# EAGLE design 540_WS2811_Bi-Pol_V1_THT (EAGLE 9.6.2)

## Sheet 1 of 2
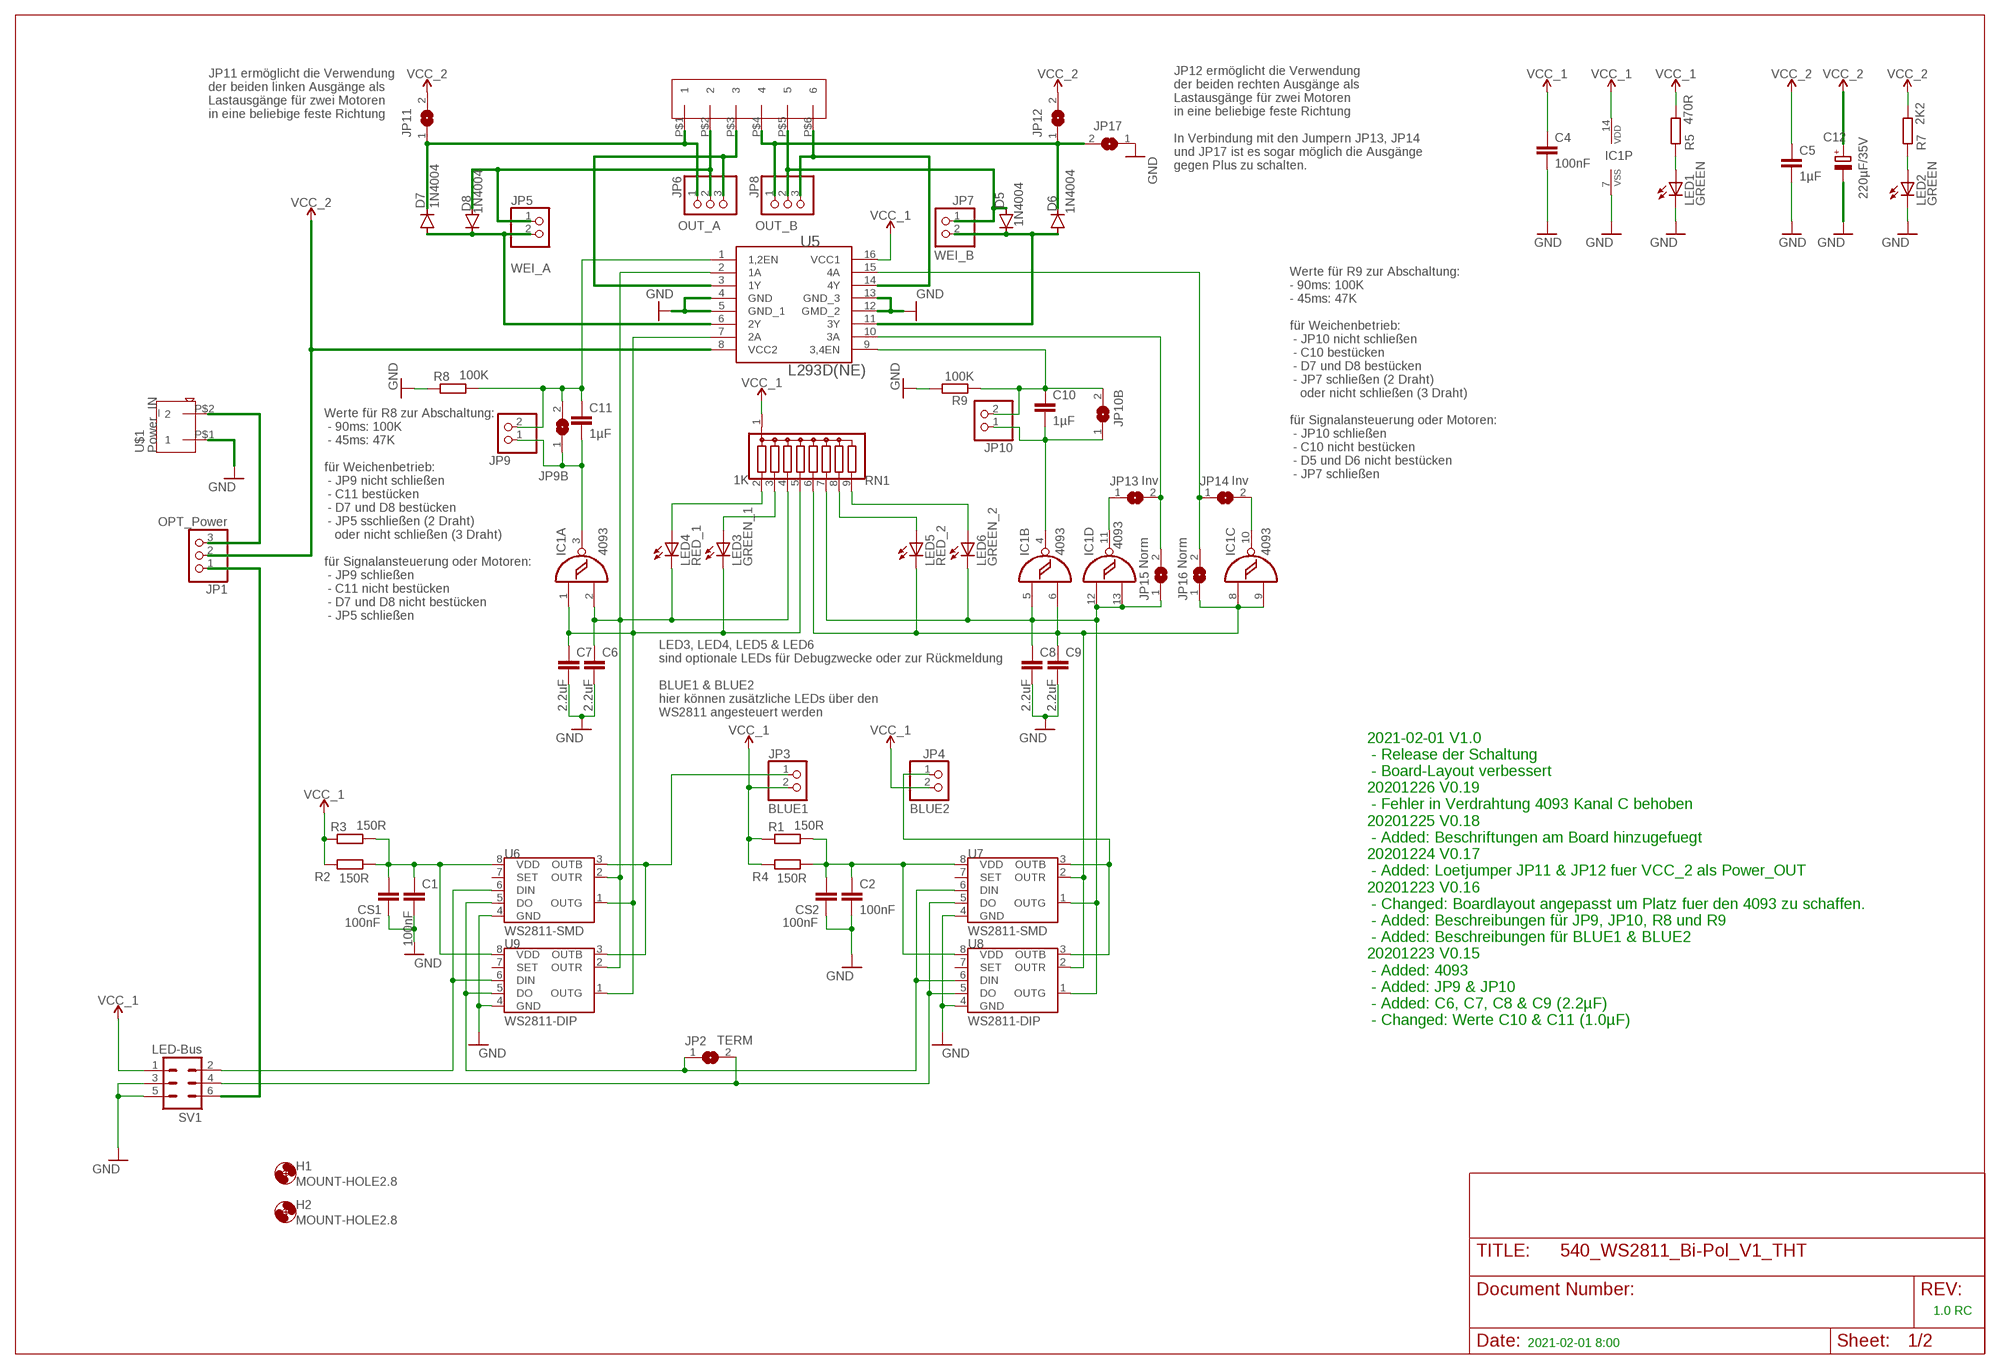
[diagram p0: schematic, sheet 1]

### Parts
C1  100nF  C-EU025-025X050  [C025-025X050]
C2  100nF  C-EU025-025X050  [C025-025X050]
C4  100nF  C-EU025-025X050  [C025-025X050]
C5  1µF  C-EU025-025X050  [C025-025X050]
C6  2.2uF  C-EU025-025X050  [C025-025X050]
C7  2.2uF  C-EU025-025X050  [C025-025X050]
C8  2.2uF  C-EU025-025X050  [C025-025X050]
C9  2.2uF  C-EU025-025X050  [C025-025X050]
C10  1µF  C-EU025-025X050  [C025-025X050]
C11  1µF  C-EU025-025X050  [C025-025X050]
C12  220µF/35V  CPOL-EUE2.5-7  [E2,5-7]
CS1  100nF  C-EUC1206  [C1206]
CS2  100nF  C-EUC1206  [C1206]
D5  1N4004  1N40041N4004-D7.5  [D-7.5]
D6  1N4004  1N40041N4004-D7.5  [D-7.5]
D7  1N4004  1N40041N4004-D7.5  [D-7.5]
D8  1N4004  1N40041N4004-D7.5  [D-7.5]
H1  MOUNT-HOLE2.8  [2,8]
H2  MOUNT-HOLE2.8  [2,8]
IC1  4093  4093N  [DIL14]
JP1  OPT_Power  PINHD-1X3  [1X03]
JP2  TERM  SJ  [SJ]
JP3  BLUE1  PINHD-1X2  [1X02]
JP4  BLUE2  PINHD-1X2  [1X02]
JP5  WEI_A  PINHD-1X2  [1X02]
JP6  OUT_A  PINHD-1X3  [1X03]
JP7  WEI_B  PINHD-1X2  [1X02]
JP8  OUT_B  PINHD-1X3  [1X03]
JP9  PINHD-1X2  [1X02]
JP9B  Inv  SJ  [SJ]
JP10  PINHD-1X2  [1X02]
JP10B  Inv  SJ  [SJ]
JP11  SJ  [SJ]
JP12  SJ  [SJ]
JP13  Inv  SJ  [SJ]
JP14  Inv  SJ  [SJ]
JP15  Norm  SJ  [SJ]
JP16  Norm  SJ  [SJ]
JP17  SJ  [SJ]
LED1  GREEN  LED3MM  [LED3MM]
LED2  GREEN  LED3MM  [LED3MM]
LED3  GREEN_1  LED3MM  [LED3MM]
LED4  RED_1  LED3MM  [LED3MM]
LED5  RED_2  LED3MM  [LED3MM]
LED6  GREEN_2  LED3MM  [LED3MM]
R1  150R  R-EU_R1206  [R1206]
R2  150R  R-EU_0207/2V  [0207/2V]
R3  150R  R-EU_R1206  [R1206]
R4  150R  R-EU_0207/2V  [0207/2V]
R5  470R  R-EU_0207/2V  [0207/2V]
R7  2K2  R-EU_0207/2V  [0207/2V]
R8  100K  R-EU_0207/2V  [0207/2V]
R9  100K  R-EU_0207/2V  [0207/2V]
RN1  1K  G08R  [SIL9]
SV1  LED-Bus  ML6  [ML6]
U5  L293D(NE)  L293DNE  [DIP-16_300MIL]
U6  WS2811-SMD  S3PO_MODUL_WS2811_SOUND_MP3-TF-16P_WS2811_AND_ATTINY_WS2811-ICSOP8  [SOP8]
U7  WS2811-SMD  S3PO_MODUL_WS2811_SOUND_MP3-TF-16P_WS2811_AND_ATTINY_WS2811-ICSOP8  [SOP8]
U8  WS2811-DIP  S3PO_MODUL_WS2811_SOUND_MP3-TF-16P_WS2811_AND_ATTINY_WS2811-ICTINY45-20-DIP  [S3PO_MODUL_WS2811_SOUND_MP3-TF-16P_WS2811_AND_ATTINY_WS2811_DIP08]
U9  WS2811-DIP  S3PO_MODUL_WS2811_SOUND_MP3-TF-16P_WS2811_AND_ATTINY_WS2811-ICTINY45-20-DIP  [S3PO_MODUL_WS2811_SOUND_MP3-TF-16P_WS2811_AND_ATTINY_WS2811_DIP08]
U$1  Power_IN  SCHRAUBKLEMME-2P  [TERM-2P]
U$2  SCHRAUBKLEMME-6P  [TERM-6P]

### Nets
GND: C1.1 C2.2 C4.2 C5.2 C6.1 C7.1 C8.1 C9.1 C12.- CS1.2 CS2.2 IC1.7(P:VSS) JP17.1 LED1.K(C) LED2.K(C) R8.1 R9.2 SV1.3 SV1.5 U5.4(GND) U5.5(GND_1) U5.12(GMD_2) U5.13(GND_3) U6.4(GND) U7.4(GND) U8.4(GND) U9.4(GND) U$1.P$1
N$1: JP1.1 SV1.6
N$2: JP1.3 U$1.P$2
N$3: C11.1 JP9.2 JP9B.2 R8.2 U5.1(1,2EN)
N$5: D6.C JP8.1 JP12.1 JP17.2 U$2.P$4
N$6: JP6.3 U5.3(1Y) U$2.P$3
N$7: D8.A JP5.1 JP6.2 U$2.P$2
N$8: JP8.3 U5.14(4Y) U$2.P$6
N$9: LED1.A R5.1
N$10: JP2.1 U6.5(DO) U7.6(DIN) U8.6(DIN) U9.5(DO)
N$11: SV1.2 U6.6(DIN) U9.6(DIN)
N$12: LED5.A RN1.8
N$13: JP3.1 U6.3(OUTB) U9.3(OUTB)
N$14: LED6.A RN1.9
N$15: C1.2 CS1.1 R2.1 R3.2 U6.8(VDD) U9.8(VDD)
N$16: JP4.1 U7.3(OUTB) U8.3(OUTB)
N$17: C2.1 CS2.1 R1.2 R4.1 U7.8(VDD) U8.8(VDD)
N$18: JP2.2 SV1.4 U7.5(DO) U8.5(DO)
N$19: C10.1 JP10.2 JP10B.2 R9.1 U5.9(3,4EN)
N$20: LED2.A R7.1
N$21: D5.C D6.A JP7.2 U5.11(3Y)
N$22: IC1.11(D:O) JP13.1
N$23: C9.2 IC1.6(B:I1) IC1.8(C:I0) IC1.9(C:I1) JP16.1 LED5.K(C) RN1.6 U7.2(OUTR) U8.2(OUTR)
N$24: C7.2 IC1.1(A:I0) LED3.K(C) RN1.5 U5.7(2A) U6.1(OUTG) U9.1(OUTG)
N$25: LED3.A RN1.3
N$26: LED4.A RN1.2
N$27: C6.2 IC1.2(A:I1) LED4.K(C) RN1.4 U5.2(1A) U6.2(OUTR) U9.2(OUTR)
N$28: D7.C JP6.1 JP11.1 U$2.P$1
N$29: D7.A D8.C JP5.2 U5.6(2Y)
N$30: C10.2 IC1.4(B:O) JP10.1 JP10B.1
N$31: D5.A JP7.1 JP8.2 U$2.P$5
N$32: C11.2 IC1.3(A:O) JP9.1 JP9B.1
N$33: C8.2 IC1.5(B:I0) IC1.12(D:I0) IC1.13(D:I1) JP15.1 LED6.K(C) RN1.7 U7.1(OUTG) U8.1(OUTG)
N$34: IC1.10(C:O) JP14.2
N$35: JP14.1 JP16.2 U5.15(4A)
N$36: JP13.2 JP15.2 U5.10(3A)
VCC_1: C4.1 IC1.14(P:VDD) JP3.2 JP4.2 R1.1 R2.2 R3.1 R4.2 R5.2 RN1.1 SV1.1 U5.16(VCC1)
VCC_2: C5.1 C12.+ JP1.2 JP11.2 JP12.2 R7.2 U5.8(VCC2)
Unconnected: U6.7(SET) U7.7(SET) U8.7(SET) U9.7(SET)

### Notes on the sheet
- JP11 ermöglicht die Verwendung 
  der beiden linken Ausgänge als
  Lastausgänge für zwei Motoren 
  in eine beliebige feste Richtung
- JP12 ermöglicht die Verwendung 
  der beiden rechten Ausgänge als
  Lastausgänge für zwei Motoren 
  in eine beliebige feste Richtung
  
  In Verbindung mit den Jumpern JP13, JP14
  und JP17 ist es sogar möglich die Ausgänge
  gegen Plus zu schalten.
- Werte für R9 zur Abschaltung:
  - 90ms: 100K
  - 45ms: 47K
  
  für Weichenbetrieb: 
   - JP10 nicht schließen
   - C10 bestücken
   - D7 und D8 bestücken
   - JP7 schließen (2 Draht) 
     oder nicht schließen (3 Draht)
  
  für Signalansteuerung oder Motoren: 
   - JP10 schließen
   - C10 nicht bestücken
   - D5 und D6 nicht bestücken
   - JP7 schließen
- Werte für R8 zur Abschaltung:
   - 90ms: 100K
   - 45ms: 47K
  
  für Weichenbetrieb: 
   - JP9 nicht schließen
   - C11 bestücken
   - D7 und D8 bestücken
   - JP5 sschließen (2 Draht) 
     oder nicht schließen (3 Draht)
  
  für Signalansteuerung oder Motoren: 
   - JP9 schließen
   - C11 nicht bestücken
   - D7 und D8 nicht bestücken
   - JP5 schließen
- LED3, LED4, LED5 & LED6 
  sind optionale LEDs für Debugzwecke oder zur Rückmeldung
  
  BLUE1 & BLUE2
  hier können zusätzliche LEDs über den
  WS2811 angesteuert werden
- 2021-02-01 V1.0
   - Release der Schaltung
   - Board-Layout verbessert
  20201226 V0.19
   - Fehler in Verdrahtung 4093 Kanal C behoben
  20201225 V0.18
   - Added: Beschriftungen am Board hinzugefuegt
  20201224 V0.17
   - Added: Loetjumper JP11 & JP12 fuer VCC_2 als Power_OUT
  20201223 V0.16
   - Changed: Boardlayout angepasst um Platz fuer den 4093 zu schaffen.
   - Added: Beschreibungen für JP9, JP10, R8 und R9
   - Added: Beschreibungen für BLUE1 & BLUE2
  20201223 V0.15
   - Added: 4093
   - Added: JP9 & JP10
   - Added: C6, C7, C8 & C9 (2.2µF)
   - Changed: Werte C10 & C11 (1.0µF)
- 1.0 RC
- 2021-02-01 8:00

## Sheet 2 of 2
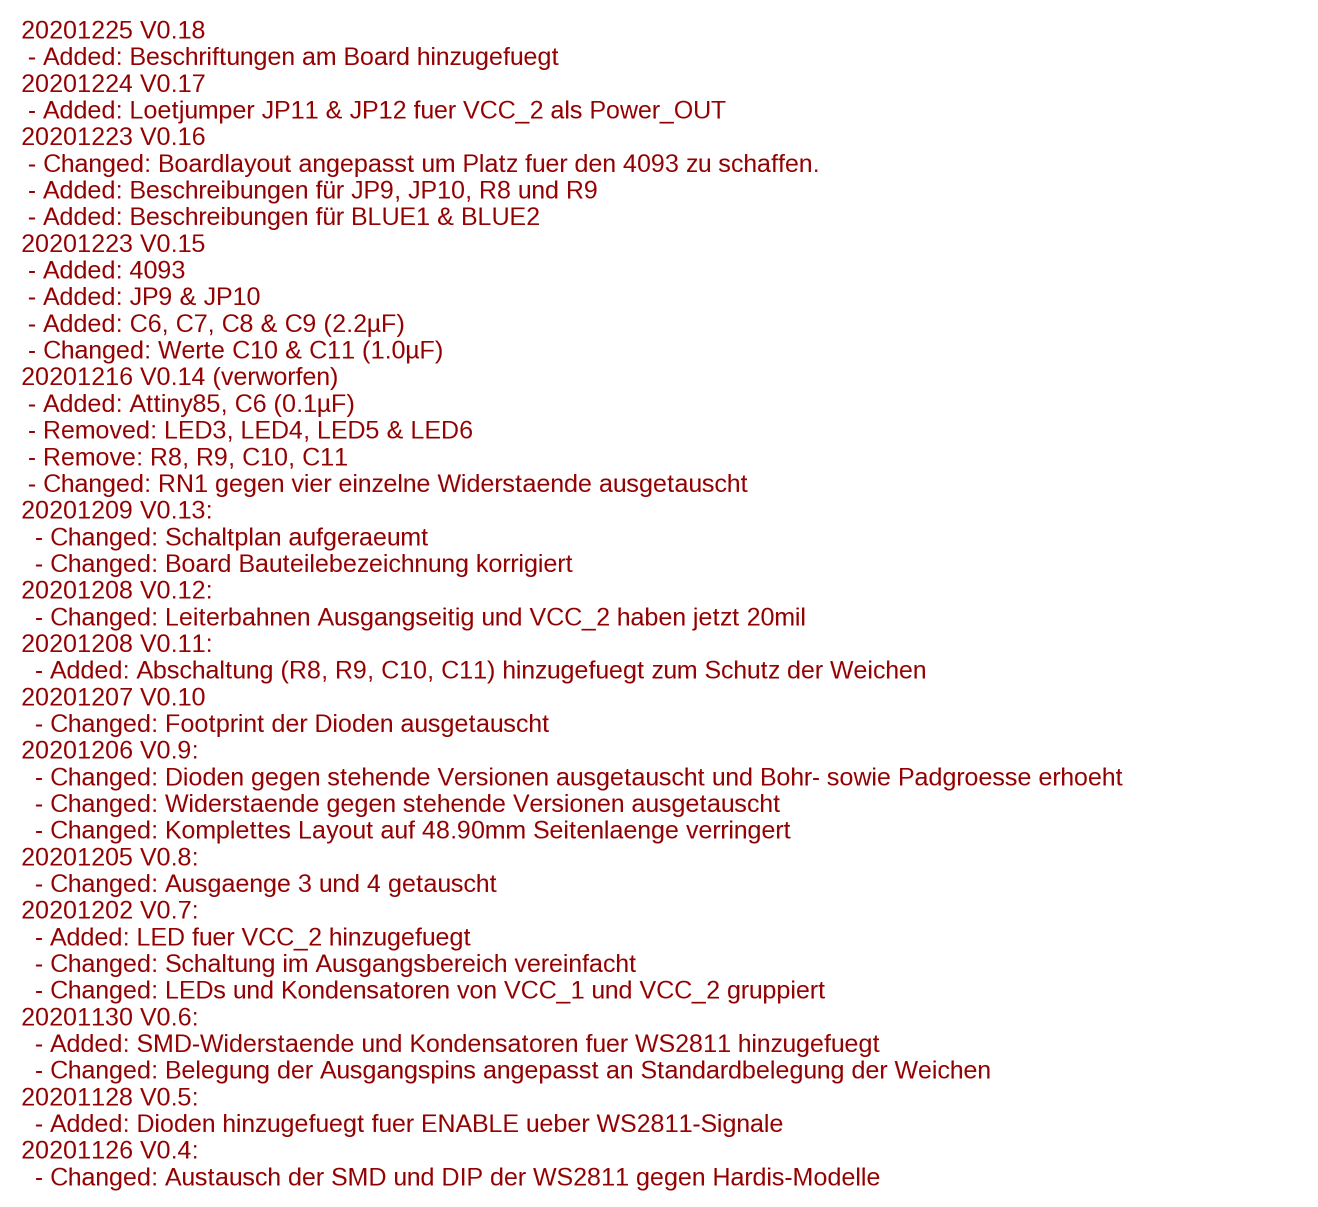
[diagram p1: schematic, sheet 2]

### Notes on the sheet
- 20201225 V0.18
   - Added: Beschriftungen am Board hinzugefuegt
  20201224 V0.17
   - Added: Loetjumper JP11 & JP12 fuer VCC_2 als Power_OUT
  20201223 V0.16
   - Changed: Boardlayout angepasst um Platz fuer den 4093 zu schaffen.
   - Added: Beschreibungen für JP9, JP10, R8 und R9
   - Added: Beschreibungen für BLUE1 & BLUE2
  20201223 V0.15
   - Added: 4093
   - Added: JP9 & JP10
   - Added: C6, C7, C8 & C9 (2.2µF)
   - Changed: Werte C10 & C11 (1.0µF)
  20201216 V0.14 (verworfen)
   - Added: Attiny85, C6 (0.1µF)
   - Removed: LED3, LED4, LED5 & LED6
   - Remove: R8, R9, C10, C11
   - Changed: RN1 gegen vier einzelne Widerstaende ausgetauscht
  20201209 V0.13:
    - Changed: Schaltplan aufgeraeumt
    - Changed: Board Bauteilebezeichnung korrigiert
  20201208 V0.12:
    - Changed: Leiterbahnen Ausgangseitig und VCC_2 haben jetzt 20mil
  20201208 V0.11:
    - Added: Abschaltung (R8, R9, C10, C11) hinzugefuegt zum Schutz der Weichen
  20201207 V0.10
    - Changed: Footprint der Dioden ausgetauscht
  20201206 V0.9:
    - Changed: Dioden gegen stehende Versionen ausgetauscht und Bohr- sowie Padgroesse erhoeht
    - Changed: Widerstaende gegen stehende Versionen ausgetauscht
    - Changed: Komplettes Layout auf 48.90mm Seitenlaenge verringert
  20201205 V0.8:
    - Changed: Ausgaenge 3 und 4 getauscht
  20201202 V0.7:
    - Added: LED fuer VCC_2 hinzugefuegt
    - Changed: Schaltung im Ausgangsbereich vereinfacht
    - Changed: LEDs und Kondensatoren von VCC_1 und VCC_2 gruppiert
  20201130 V0.6:
    - Added: SMD-Widerstaende und Kondensatoren fuer WS2811 hinzugefuegt
    - Changed: Belegung der Ausgangspins angepasst an Standardbelegung der Weichen
  20201128 V0.5: 
    - Added: Dioden hinzugefuegt fuer ENABLE ueber WS2811-Signale
  20201126 V0.4: 
    - Changed: Austausch der SMD und DIP der WS2811 gegen Hardis-Modelle

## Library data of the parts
C1 C2 C4-C11 CS1 CS2 = rcl:C-EU: CAPACITOR, European symbol; SPICEPREFIX: C
C12 = rcl:CPOL-EU: POLARIZED CAPACITOR, European symbol; SPICEPREFIX: C
D5-D8 = DH_diode:1N4004: DIODE
H1 H2 = holes:MOUNT-HOLE: MOUNTING HOLE with drill center marker
IC1 = 40xx:4093: Quad 2-input NAND schmitt trigger
JP1 JP6 JP8 = Connector:PINHD-1X3: PIN HEADER; CATEGORY: CONNECTOR; SUB-CATEGORY: PIN-HEADER
JP2 JP9B JP10B JP11-JP17 = jumper:SJ: SMD solder JUMPER
JP3-JP5 JP9 JP10 = Connector:PINHD-1X2: PIN HEADER; CATEGORY: CONNECTOR; SUB-CATEGORY: PIN-HEADER
JP7 = pinhead:PINHD-1X2: PIN HEADER
LED1-LED6 = adafruit:LED: LED
R1-R5 R7-R9 = rcl:R-EU_: RESISTOR, European symbol; SPICEPREFIX: R
RN1 = resistor-sil:G08R: SIL RESISTOR; OC_FARNELL: unknown; OC_NEWARK: unknown
SV1 = con-ml:ML6: HARTING; OC_FARNELL: unknown; OC_NEWARK: unknown
U5 = IC:L293DNE: IC MTR DRV BIPOLAR 4.5-36V 16DIP Manufacturer's datasheet; CREATED_BY: PCBLayout.com; DIGI-KEY_PART: 296-9518-5-ND; MANUFACTURER: Texas Instruments; MPN: L293DNE; PACKAGE: DIP-16
U6 U7 = S3PO_Modul_WS2811:S3PO_MODUL_WS2811_SOUND_MP3-TF-16P_WS2811_AND_ATTINY_WS2811-IC: Die Pin Nummern für R und G sind getauscht damit sie gleich angesteuert werden wie die WS2812. Der Daten Strom der WS2811 ist RGB, Beim WS2812 ist es aber GRB.
U8 U9 = S3PO_Modul_WS2811:S3PO_MODUL_WS2811_SOUND_MP3-TF-16P_WS2811_AND_ATTINY_WS2811-IC: Die Pin Nummern für R und G sind getauscht damit sie gleich angesteuert werden wie die WS2812. Der Daten Strom der WS2811 ist RGB, Beim WS2812 ist es aber GRB.; PROD_ID: IC-09439; VALUE: TINY45-20-DIP
U$1 = MLL-Dominik-Hardi:SCHRAUBKLEMME-2P
U$2 = MLL-Dominik-Hardi:SCHRAUBKLEMME-6P

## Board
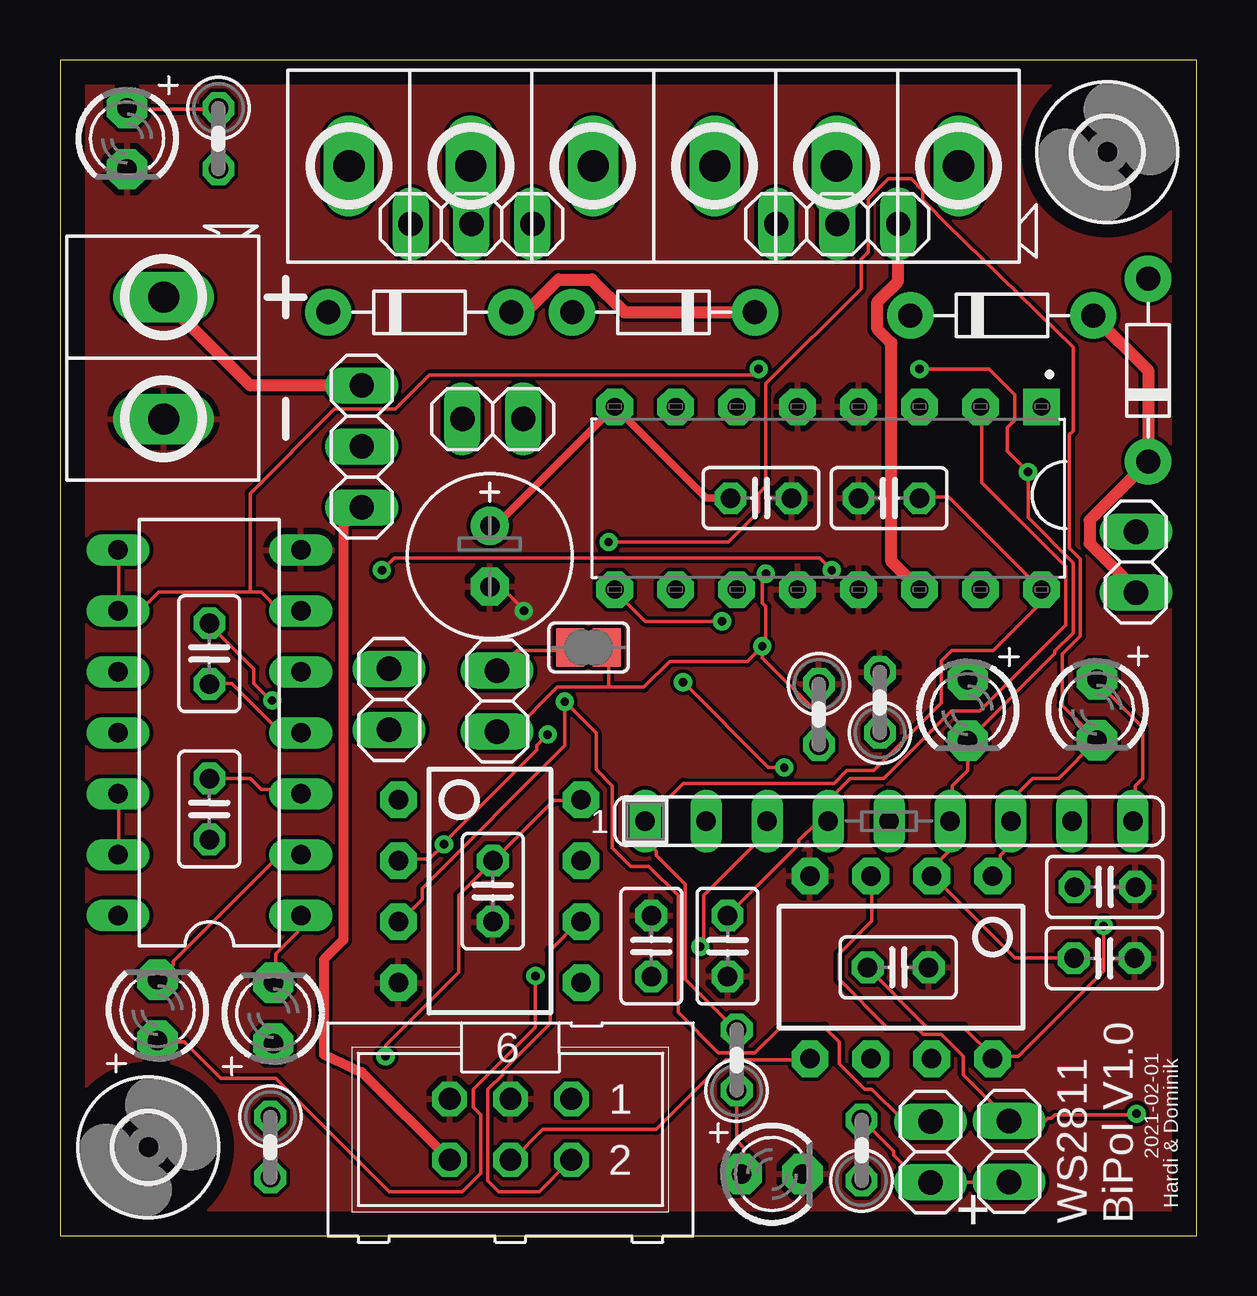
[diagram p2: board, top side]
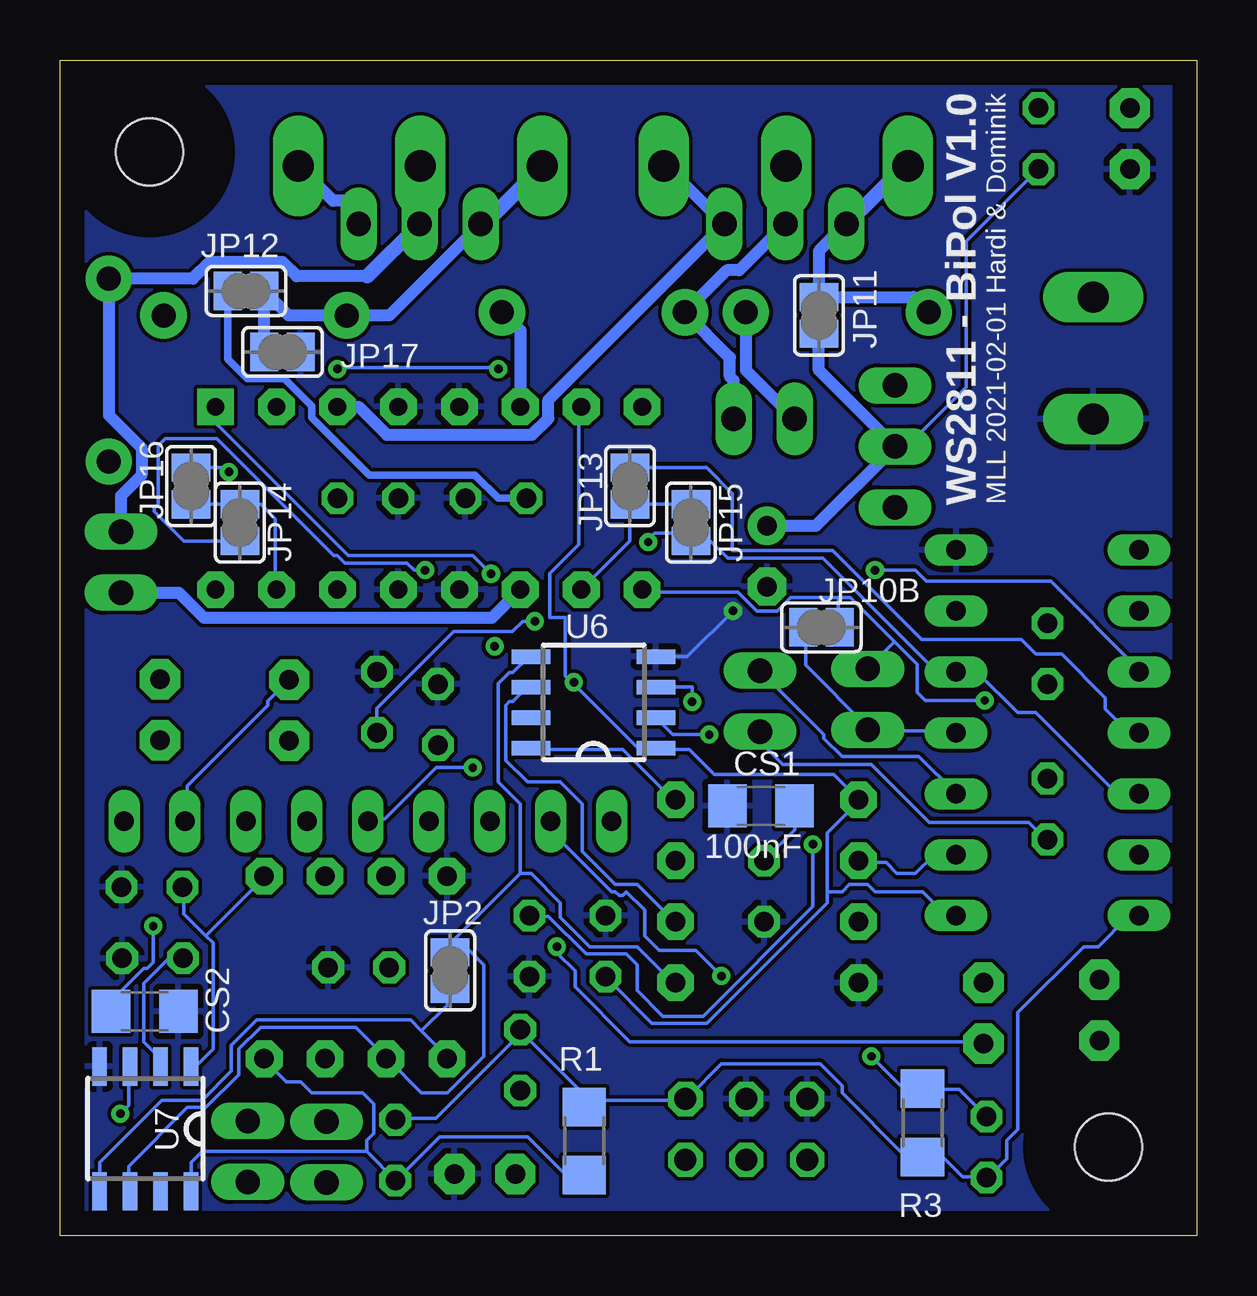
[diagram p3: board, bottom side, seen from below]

Size 47.37 x 49 mm. Coordinates in mm from the lower left corner, seen from the top.
Outline: 0,0 47.37,0 47.37,49 0,49 0,0
Copper layers (1*16): Top 0.035mm / dielectric 1.5mm / Bottom 0.035mm
Design rules "default": minimum track width 6mil, minimum drill 0.35mm, track to track 6mil, track to pad 6mil, pad to pad 6mil, via to via 6mil, smd to smd 6mil, copper to edge 40mil, drill to drill 6mil, minimum pad ring 10mil, minimum via ring 8mil, stop-mask expansion 4mil, vias tented up to drill 0mil, thermal gap 10mil

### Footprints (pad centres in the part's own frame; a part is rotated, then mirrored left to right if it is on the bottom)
C025-025X050 = drill 0.813 octagon: 1 -1.27,0; 2 1.27,0
E2,5-7 = drill 0.813 pad 1.6: + -1.27,0 | drill 0.813 pad 1.6 octagon: - 1.27,0
C1206 = smd 1.6 x 1.8: 1 -1.4,0; 2 1.4,0
D-7.5 = drill 1 pad 1.93: A 3.81,0; C -3.81,0
2,8 = hole 2.8: 0,0
DIL14 = drill 0.813 long: 1 -7.62,-3.81; 2 -5.08,-3.81; 3 -2.54,-3.81; 4 0,-3.81; 5 2.54,-3.81; 6 5.08,-3.81; 7 7.62,-3.81; 8 7.62,3.81; 9 5.08,3.81; 10 2.54,3.81; 11 0,3.81; 12 -2.54,3.81; 13 -5.08,3.81; 14 -7.62,3.81
1X03 = drill 1.016 long: 1 -2.54,0; 2 0,0; 3 2.54,0
SJ = smd 1.168 x 1.6: 1 -0.762,0; 2 0.762,0
1X02 = drill 1.016 long: 1 -1.27,0; 2 1.27,0
LED3MM = drill 0.813 pad 1.676 octagon: A -1.27,0; K 1.27,0
R1206 = smd 1.6 x 1.803: 1 -1.422,0; 2 1.422,0
0207/2V = drill 0.813 octagon: 1 -1.27,0; 2 1.27,0
SIL9 = drill 0.813 long: 1 -10.16,0; 2 -7.62,0; 3 -5.08,0; 4 -2.54,0; 5 0,0; 6 2.54,0; 7 5.08,0; 8 7.62,0; 9 10.16,0
ML6 = drill 0.914 octagon: 1 -2.54,-1.27; 2 -2.54,1.27; 3 0,-1.27; 4 0,1.27; 5 2.54,-1.27; 6 2.54,1.27
DIP-16_300MIL = drill 0.74 pad 1.524 square: 1 -3.81,8.89 | drill 0.74 pad 1.524 octagon: 2 -3.81,6.35; 3 -3.81,3.81; 4 -3.81,1.27; 5 -3.81,-1.27; 6 -3.81,-3.81; 7 -3.81,-6.35; 8 -3.81,-8.89; 9 3.81,-8.89; 10 3.81,-6.35; 11 3.81,-3.81; 12 3.81,-1.27; 13 3.81,1.27; 14 3.81,3.81; 15 3.81,6.35; 16 3.81,8.89
SOP8 = smd 0.6 x 1.6: 1 -1.905,-2.6; 2 -0.635,-2.6; 3 0.635,-2.6; 4 1.905,-2.6; 5 1.905,2.6; 6 0.635,2.6; 7 -0.635,2.6; 8 -1.905,2.6
S3PO_MODUL_WS2811_SOUND_MP3-TF-16P_WS2811_AND_ATTINY_WS2811_DIP08 = drill 0.813 pad 1.524 octagon: 1 -3.81,-3.81; 2 -1.27,-3.81; 3 1.27,-3.81; 4 3.81,-3.81; 5 3.81,3.81; 6 1.27,3.81; 7 -1.27,3.81; 8 -3.81,3.81
TERM-2P = drill 1.3 pad 2.1 long: P$1 -2.54,0; P$2 2.54,0
TERM-6P = drill 1.3 pad 2.1 long: P$1 -12.6,0.26; P$2 -7.52,0.26; P$3 -2.42,0.26; P$4 2.64,0.26; P$5 7.72,0.26; P$6 12.8,0.26

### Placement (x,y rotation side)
C1  18.03,14.35 90 top
C2  34.92,11.18 0 top
C4  34.54,30.73 180 top
C5  29.21,30.73 0 top
C6  27.81,12.06 90 top
C7  24.64,12.06 270 top
C8  43.54,14.53 180 top
C9  43.51,11.56 180 top
C10  6.22,24.26 270 top
C11  6.22,17.78 90 top
C12  17.91,28.32 270 top
CS1  18.16,17.91 180 bottom
CS2  43.84,9.35 0 bottom
D5  45.34,36.07 90 top
D6  39.24,38.35 0 top
D7  14.99,38.48 0 top
D8  25.15,38.48 180 top
H1  3.68,3.68 0 top
H2  43.64,45.16 0 top
IC1  6.22,20.95 90 top
JP1  12.57,32.89 90 top
JP2  31.11,11.05 270 bottom
JP3  36.27,3.48 270 top
JP4  39.55,3.51 270 top
JP5  18.03,34.04 180 top
JP6  17.14,42.16 0 top
JP7  44.83,28.07 270 top
JP8  32.38,42.16 0 top
JP9  18.21,22.28 270 top
JP9B  22.02,24.51 0 top
JP10  13.72,22.35 90 top
JP10B  15.65,25.35 0 bottom
JP11  15.75,38.35 270 bottom
JP12  39.62,39.37 180 bottom
JP13  23.62,31.24 270 bottom
JP14  39.88,29.72 270 bottom
JP15  21.08,29.72 90 bottom
JP16  41.91,31.24 270 bottom
JP17  38.1,36.83 180 bottom
LED1  29.67,2.57 0 top
LED2  2.79,45.72 270 top
LED3  8.89,9.27 90 top
LED4  4.06,9.4 90 top
LED5  37.82,21.89 270 top
LED6  43.21,21.92 270 top
R1  25.53,3.94 270 bottom
R2  8.76,3.68 270 top
R3  11.43,4.7 90 bottom
R4  33.4,3.56 90 top
R5  28.19,7.32 90 top
R7  6.6,45.72 270 top
R8  31.62,21.72 270 top
R9  34.16,22.23 90 top
RN1  34.54,17.27 0 top
SV1  18.77,4.42 180 top
U5  32,30.73 270 top
U6  25.15,22.23 90 bottom
U7  43.81,4.45 180 bottom
U8  35.05,11.18 180 top
U9  17.91,14.35 270 top
U$1  4.32,36.58 90 top
U$2  24.64,44.32 0 top

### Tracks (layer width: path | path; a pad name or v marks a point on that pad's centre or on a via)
GND  (via drill 0.35)
  Top 0.152: C12.- 18.36,27.05 19.36,26.06 v19.33,26.04
  Bottom 0.152: v19.33,26.04 21.23,24.13 U6.4
  pour Bottom: 0.51,48.51 0.51,0.25 46.99,0.25 46.99,48.51
  pour Top: 0.51,48.51 0.51,0.25 46.99,0.25 46.99,48.51
N$1
  Top 0.305: 11,7.92 11,7.54
  Top 0.406: JP1.1 11.81,29.59 11.81,27.94 11.81,12.32 11,11.51 11,7.92 11,7.54 12.57,6.81 SV1.6
N$2
  Top 0.152: 4.27,39.09 U$1.P$2
  Top 0.508: JP1.3 7.93,35.43 4.27,39.09
N$3  (via drill 0.35)
  Top 0.152: v29.41,27.58 29.26,27.43 29.26,26.36 29.41,26.21 29.41,24.71 v29.26,24.56 29.26,24.54 | 29.26,24.54 29.23,24.54 28.63,23.93 26.31,23.93 25.4,23.93 24.33,22.86 22.86,22.86 | 22.86,22.86 20.75,22.86 20.73,22.86 18.9,21.03 18.29,21.03 JP9.2 | 29.26,24.54 29.26,24.08 31.55,21.79 31.55,20.57 R8.2 | 22.86,22.86 22.86,24.38 JP9B.2
  Bottom 0.152: C11.1 6.25,16.46 7.01,17.22 11.15,17.22 13.56,19.63 17.25,19.63 18.16,20.55 18.14,20.57 18.14,20.88 JP9.2 | v29.41,27.58 30.18,28.35 35.36,28.35 40.84,33.83 40.84,34.44 U5.1
N$5
  Bottom 0.508: 38.73,39.24 37.85,38.35 D6.C 33.66,38.35 JP8.1 29.84,42.91 | 38.73,39.24 JP12.1 | JP17.2 38.86,39.12 38.73,39.24
  Bottom 0.61: U$2.P$4 29.7,42.16 JP8.1 29.84,42.91
N$6
  Bottom 0.508: U5.3 34.93,34.54 33.76,33.38 27.71,33.38 27.03,34.06 27.03,34.82 19.94,41.91 JP6.3 22.1,44.58 U$2.P$3
N$7
  Bottom 0.508: U$2.P$2 17.12,45.57 17.14,45.59 JP6.2 19.07,40.23 19.58,40.23 D8.A 19.46,36.6 19.46,35.79 19.3,35.64 JP5.1
N$8
  Top 0.508: JP8.3 34.92,39.79 34.06,38.92 34.06,37.79 34.65,37.2 34.65,28.09 U5.14
  Bottom 0.508: U$2.P$6 35.99,43.13 35.1,43.13
  Bottom 0.61: JP8.3 34.92,42.96 35.1,43.13
N$9
  Top 0.152: R5.1 28.19,3.96 28.5,3.66 28.5,2.59 LED1.A
N$10
  Bottom 0.152: U7.6 44.5,1.98 44.5,2.9 42.06,5.33 41.3,5.33 39.93,6.71 39.93,7.77 39.01,8.69 35.05,8.69 33.83,7.47 U8.6 33.68,7.32 32.31,5.94 31.24,5.94 29.72,7.47 29.72,11.28 30.33,11.89 31.09,11.89 | 28.19,15.09 31.09,12.19 31.09,11.89 | 28.19,15.09 27.74,15.09 26.52,13.87 26.52,13.26 25.3,12.04 23.32,12.04 22.25,10.97 22.1,10.97 21.79,10.67 U9.5 | 31.09,11.89 JP2.1 | 28.19,15.09 28.19,17.98 29.11,18.9 29.11,23.01 28.65,23.47 28.5,23.47 27.89,24.08 U6.5
N$11
  Top 0.152: SV1.2 21.18,3.05 19.96,1.83 18.29,1.83 17.83,2.29 17.83,6.1 18.44,6.71 18.44,6.86 20.42,8.84 20.42,11.89 21.64,13.11 U9.6
  Bottom 0.152: U9.6 21.79,13.11 23.32,14.63 24.23,14.63 25.6,16 25.6,17.98 26.52,18.9 27.89,18.9 28.8,19.81 28.8,22.1 28.65,22.25 28.5,22.25 27.89,22.86 U6.6
N$12
  Bottom 0.152: RN1.8 42.06,17.37 42.06,18.75 38.71,22.1 38.71,22.28 LED5.A
N$13  (via drill 0.35)
  Top 0.152: U9.3 14.17,13.11 15.09,14.02 15.09,14.48 21.03,20.42 v21.03,22.25 22.34,20.94 22.34,19.42 23.01,18.75 23.01,16.15 23.77,15.39 24.54,15.39 25.76,14.17 25.76,9.3 27.43,7.62 28.96,7.62 30.02,8.69 31.85,8.69 32.46,8.08 32.46,7.16 33.53,6.1 33.83,6.1 35.05,4.88 36.08,4.88 JP3.1
  Bottom 0.152: U6.3 21.03,22.86 v21.03,22.25
N$14
  Top 0.152: RN1.9 44.81,17.37 44.81,18.75 45.11,19.05 45.11,21.18 43.13,23.16 LED6.A
N$15  (via drill 0.35)
  Top 0.152: U9.8 21.64,18.14 20.57,18.14 18.14,15.7 C1.2 17.98,15.54 16.61,14.17 16.61,10.97 13.56,7.92 v13.56,7.47
  Bottom 0.152: R2.1 9.91,6.1 11.43,6.1 R3.2 11.43,6.25 12.34,6.25 v13.56,7.47 | CS1.1 16.76,17.83 16.76,16.92 17.98,15.7 C1.2 | U6.8 27.71,20.27 23.93,20.27 21.79,18.14 U9.8
N$16  (via drill 0.35)
  Top 0.152: v44.86,5.08 44.91,5.03 41.45,5.03 41.3,4.88 41.15,4.88 41,4.72 39.62,4.72 39.57,4.78 | 39.57,4.78 37.64,6.71 37.64,7.47 36.73,8.38 35.97,8.38 35.66,8.69 34.44,8.69 32.46,10.67 32.46,11.73 33.83,13.11 33.83,14.94 U8.3 | 39.57,4.78 JP4.1
  Bottom 0.152: v44.86,5.08 44.5,5.44 44.5,7.01 U7.3
N$17  (via drill 0.35)
  Top 0.152: v43.48,12.9 43.48,11.02 39.93,7.47 38.86,7.47 | 38.86,7.47 37.64,8.69 36.12,8.69 33.68,11.12 C2.1 | 38.86,7.47 U8.8
  Bottom 0.152: U7.8 41.91,3.05 41.45,3.5 34.59,3.5 | 33.38,2.29 34.59,3.5 | 33.38,2.29 31.55,4.12 27.89,4.12 26.36,2.59 25.6,2.59 R1.2 | 33.38,2.29 R4.1 | v43.48,12.9 43.48,11.38 43.74,11.12 43.89,11.12 45.11,9.91 45.11,9.45 CS2.1 | 34.59,3.5 34.59,3.96 34.29,4.27 34.29,5.49 34.75,5.94 36.88,5.94 37.34,6.4 37.95,6.4 38.86,7.32 U8.8
N$18
  Top 0.152: SV1.4 18.9,3.2 20.12,4.42 24.84,4.42 27.74,7.32 31.24,7.32 U8.5
  Bottom 0.152: U7.5 45.72,3.05 43.13,5.64 41.45,5.64 40.23,6.86 40.23,7.92 39.17,8.99 32.77,8.99 32.31,8.53 | 32.31,8.53 31.24,7.47 U8.5 | 32.31,8.53 31.24,9.6 31.24,10.21 JP2.2
N$19  (via drill 0.35)
  Top 0.152: v8.84,22.3 8.79,22.3 8.08,23.01 8.08,23.62 6.25,25.45 C10.1 | v27.58,25.6 24.38,25.6 23.16,26.82 U5.9
  Bottom 0.152: U5.9 23.01,26.82 19.13,26.82 18.33,26.02 17.48,26.02 16.91,26.59 14.94,26.59 | v8.84,22.3 11.33,22.3 11.66,22.63 11.66,23.8 12.6,24.74 | R9.1 34.16,21.97 30.96,25.17 28.52,25.17 28.09,25.6 v27.58,25.6 | 14.94,26.59 14.45,26.59 12.6,24.74 | JP10B.2 14.94,25.45 14.94,26.52 14.94,26.59 | JP10.2 12.65,24.69 12.6,24.74
N$20
  Top 0.152: R7.1 6.55,46.94 2.9,46.94 LED2.A
N$21
  Top 0.508: D6.A 45.34,36.07 D5.C 43.59,30.5 42.9,29.82 42.9,28.85 44.83,26.92 JP7.2
  Bottom 0.508: JP7.2 42.42,26.8 41.38,25.76 29.36,25.76 U5.11
N$22
  Bottom 0.152: JP13.1 20.42,32 19.36,30.94 19.36,28.55 15.16,28.55 11.46,24.84 7.32,24.84 6.71,24.23 5.64,24.23 3.81,22.4 3.81,21.95 2.9,21.03 2.44,21.03 IC1.11
N$23  (via drill 0.35)
  Top 0.152: 2.44,26.36 2.44,28.5 IC1.8 | 2.44,26.36 2.44,26.06 IC1.9 2.44,26.36 | 7.92,26.82 4.12,26.82 3.66,26.36 2.44,26.36 | 7.92,26.82 8.38,26.82 9.14,26.06 9.91,26.06 IC1.6 | C9.2 42.22,11.58 39.78,11.58 36.42,14.94 U8.2 36.42,15.09 36.42,15.39 37.03,16 37.03,17.22 RN1.6 37.19,17.37 37.19,18.75 37.72,19.28 37.82,19.38 LED5.K 41.45,24.26 41.45,24.36 42.22,25.12 42.22,28.04 40.34,29.92 v40.34,31.83 39.47,32.69 39.47,33.68 39.78,33.98 39.78,35.05 38.71,36.12 v35.81,36.12 | 7.92,26.82 7.92,30.94 11.43,34.44 13.97,34.44 15.39,35.87 28.85,35.87 v29.11,36.12
  Bottom 0.152: U7.2 43.28,7.16 43.28,7.47 43.89,8.08 43.89,10.52 42.82,11.58 42.37,11.58 C9.2 | JP16.1 40.51,32 v40.34,31.83 | v29.11,36.12 29.16,36.17 35.76,36.17 v35.81,36.12
N$24  (via drill 0.35)
  Top 0.152: IC1.1 9.91,13.26 9.91,12.65 8.99,11.73 8.99,10.67 LED3.K | v30.18,19.51 29.52,19.51 v25.96,23.06
  Bottom 0.152: 14.05,18.14 15.14,19.23 20.12,19.23 21.16,20.27 22.53,20.27 U6.1 23.31,20.32 26.04,23.05 | 15.39,14.33 15.39,16.79 14.05,18.14 | 15.39,14.33 15.39,13.87 20.42,8.84 22.71,8.84 24.54,10.67 C7.2 | U9.1 14.07,18.16 14.05,18.14 | 26.04,23.05 26.31,23.33 26.31,25.76 26.98,25.76 26.98,27.58 25.76,28.8 25.76,34.44 U5.7 | 15.39,14.33 14.78,14.33 14.48,14.63 13.72,14.63 13.41,14.33 11.43,14.33 10.52,13.41 10.06,13.41 IC1.1 | v30.18,19.51 31.7,19.51 33.83,17.37 34.44,17.37 RN1.5 | v25.96,23.06 26.04,23.05
N$25  (via drill 0.35)
  Top 0.152: v26.67,12.04 26.82,12.19 26.82,14.17 29.41,16.76 29.41,17.22 RN1.3
  Bottom 0.152: v26.67,12.04 26.67,11.79 25.91,11.02 25.91,10.36 23.62,8.08 8.99,8.08 LED3.A
N$26  (via drill 0.35)
  Top 0.152: v19.81,10.82 19.81,8.69 17.22,6.1 17.22,5.33 17.53,5.03 17.53,2.59 16.76,1.83 13.72,1.83 8.99,6.55 6.71,6.55 5.18,8.08 4.12,8.08 LED4.A
  Bottom 0.152: v19.81,10.82 20.88,11.89 22.4,11.89 23.01,12.5 23.01,13.56 23.77,14.33 23.93,14.17 24.08,14.17 24.23,14.33 24.38,14.33 26.82,16.76 26.82,17.22 RN1.2
N$27  (via drill 0.35)
  Top 0.152: v20.32,20.88 19.86,20.42 19.86,20.24 15.96,16.34 v16,16.31 15.39,15.7 14.17,15.7 U9.2 | LED4.K 4.12,10.67 4.72,11.28 4.72,11.43 9.14,15.85 9.91,15.85 IC1.2 | C6.2 30.79,16.31 30.79,16.46 31.55,17.22 32,17.22 RN1.4 32,18.14 32.92,19.05 34.31,19.05 37.13,21.87 38.33,21.87 41.91,25.45 41.91,27.89 38.41,31.39 38.41,34.44 U5.2
  Bottom 0.152: U6.2 21.84,20.88 v20.32,20.88 | IC1.2 10.06,15.85 10.97,15.85 11.73,15.09 12.5,15.09 12.95,15.54 14.02,15.54 U9.2 | v16,16.31 16,13.72 20.57,9.14 22.25,9.14 23.32,10.21 23.32,11.28 23.77,11.73 25.45,11.73 27.03,13.31 27.79,13.31 C6.2
N$28
  Bottom 0.508: JP6.1 15.75,41.02 JP11.1 11.81,39.12 D7.C
  Bottom 0.61: U$2.P$1 12.16,44.58 13.97,42.78 13.99,42.78 JP6.1
N$29
  Top 0.508: D7.A 19.4,38.48 20.77,39.85 22.16,39.85 23.53,38.48 D8.C
  Bottom 0.508: D7.A 18.8,36.07 JP5.2 | D8.C 28.19,37.72 U5.6
N$30
  Top 0.152: C10.2 6.25,23.01 7.16,23.01 9.14,21.03 9.91,21.03 IC1.4
  Bottom 0.152: 10.06,21.03 IC1.4 10.06,21.03 | JP10B.1 16.31,25.3 16.31,23.77 13.72,21.18 JP10.1 13.72,21.03 10.06,21.03
N$31
  Bottom 0.508: 34.57,39.98 37.51,39.98 38.11,40.58 41.14,40.58 41.84,39.88 D5.A 45.34,34.2 43.97,32.83 43.97,31.69 44.83,30.83 JP7.1
  Bottom 0.61: U$2.P$5 32.36,42.19 JP8.2 34.57,39.98
N$32
  Top 0.152: C11.2 7.92,19.05 8.38,18.59 9.75,18.59 9.91,18.44 IC1.3 | JP9B.1 21.18,24.38 19.05,24.38 18.29,23.62 JP9.1
  Bottom 0.152: IC1.3 10.06,18.44 11.58,19.96 14.78,19.96 15.54,20.73 15.54,20.88 18.14,23.47 JP9.1
N$33  (via drill 0.35)
  Top 0.152: U8.1 38.86,15.09 39.17,15.39 39.17,15.85 39.62,16.31 RN1.7 39.62,18.14 40.54,19.05 41.6,19.05 LED6.K 41.76,22.1 41.76,24.23 42.52,24.99 42.52,28.19 42.06,28.65 42.06,33.38 42.22,33.53 42.22,37.03 36.96,42.16 36.07,43.05 35.94,43.18 35.94,43.56 35.46,44.04 35.2,44.04 34.52,44.04 33.68,43.2 33.68,41 33.38,40.69 33.38,39.47 29.41,35.51 29.41,35.2 29.41,31.55 29.39,31.52 29.39,31.22 29.11,30.94 29.11,30.18 27.84,28.91 v22.86,28.91 | IC1.13 2.44,16 2.44,18.29 IC1.12
  Bottom 0.152: 41.3,12.5 42.22,13.41 42.22,14.48 C8.2 | 41.3,12.5 41,12.19 41,7.77 41.6,7.16 41.91,7.16 U7.1 | 41.3,12.5 38.86,14.94 U8.1 | IC1.12 2.44,18.44 3.35,18.44 6.71,21.79 7.47,21.79 9.14,23.47 9.91,23.47 IC1.5 10.06,23.62 10.97,23.62 15.6,28.25 19.56,28.25 20.27,28.96 JP15.1 21.18,28.96 21.51,29.29 22.58,29.29 22.86,29.01 v22.86,28.91
N$34  (via drill 0.35)
  Top 0.152: v32.16,27.74 31.65,28.25 13.92,28.25 v13.41,27.74
  Bottom 0.152: JP14.2 42.22,28.96 43.43,30.18 43.43,30.33 43.28,30.48 43.28,32.92 42.98,33.22 40.84,33.22 35.97,28.35 35.81,28.35 35.51,28.04 32.92,28.04 32.61,27.74 v32.16,27.74 | v13.41,27.74 11.73,27.74 11.28,27.28 6.1,27.28 2.44,23.62 IC1.10
N$35
  Bottom 0.152: JP16.2 JP14.1 39.01,30.48 38.41,29.87 38.41,26.98 U5.15
N$36
  Bottom 0.152: JP15.2 JP13.2 23.62,28.96 U5.10
VCC_1
  Top 0.152: C4.1 35.81,30.79 37.03,30.79 U5.16 40.89,26.39 38.89,24.38 37.16,24.38 36.73,23.95 36.73,22.2 33.91,19.38 32.79,19.38 32.26,18.85 25.96,18.85 | R4.2 33.53,4.72 34.75,3.5 34.75,3.35 35.89,2.21 JP3.2 39.53,2.21 JP4.2 | R5.2 28.19,8.53 26.06,10.67 26.06,14.63 24.84,15.85 24.84,16 24.38,16.46 RN1.1 25.88,18.77 | 25.88,18.77 25.96,18.85 | 25.88,18.77 25.96,18.85
  Bottom 0.152: IC1.14 2.44,13.26 2.9,13.26 4.12,12.04 4.72,12.04 7.47,9.3 7.47,4.42 7.92,3.96 7.92,3.2 8.69,2.44 R2.2 8.84,2.44 9.75,2.44 10.52,3.2 11.43,3.2 R3.1 11.43,3.35 12.19,3.35 14.78,5.94 14.78,6.25 15.7,7.16 19.81,7.16 21.18,5.79 SV1.1 21.34,5.64 25.6,5.64 | 25.6,5.64 25.6,5.94 28,8.34 28.13,8.47 | 25.6,5.64 25.6,5.49 R1.1 25.6,5.64 | 28.13,8.47 28.19,8.53 R5.2 | 28.13,8.47 31.73,4.88 33.38,4.88 R4.2
VCC_2
  Top 0.305: C12.+ 18.16,29.59 U5.8 26.92,30.73 C5.1
  Bottom 0.152: R7.2 9.6,41.45 9.6,35.36 12.04,32.92 12.34,32.92 JP1.2 | 40.39,38.61 JP12.2
  Bottom 0.305: C5.1 29.11,30.73 30.08,31.7 34.48,31.7 36.88,34.1 36.88,34.58 38.03,35.73 39.57,35.73 40.39,36.54 40.39,38.61
  Bottom 0.508: JP11.2 15.75,36.07 JP1.2 15.88,29.59 C12.+

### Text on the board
tPlace: 2021-02-01 / Hardi & Dominik | WS2811 / BiPol V1.0 | +
bPlace: MLL 2021-02-01 Hardi & Dominik | WS2811 - BiPol V1.0

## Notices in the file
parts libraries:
SparkFun-PowerSymbols: Licensing: Creative Commons ShareAlike 4.0 International - https://creativecommons.org/licenses/by-sa/4.0
